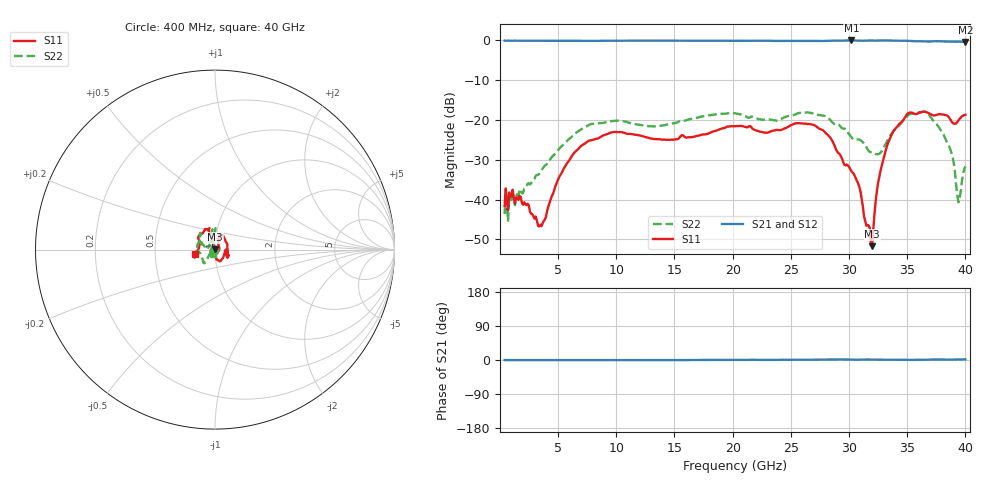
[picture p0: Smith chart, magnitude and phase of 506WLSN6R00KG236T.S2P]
!  American Technical Ceramics  Date:  8/31/2012
!  One Norden Lane
!  Huntington Station,  NY.  11746-2102
!  Tel:  (631) 622-4700  Fax:  (631) 622-4748
!  Part Number  506WLSN6R00KG236T
!  Description:  Ultra-Broadband Inductor
!  Application:  Ultra-broadband DC block decoupling, bias tee
# GHZ S DB R 50
! Freq  |S11|  S11 Ph  |S21|  S21 Ph  |S12|  S12 Ph  |S22|  S22 Ph
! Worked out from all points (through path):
!   401 points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, 400 MHz to 40 GHz, reference 50 ohm
!   highest |S21| = -0.01 dB at 30.2 GHz (marker M1); lowest = -0.4 dB at 40 GHz (marker M2)
!   lowest |S11| = -51.7 dB at 31.98 GHz (marker M3), VSWR 1.01, Z = 50.1 + j0.216 ohm
!   |S11| at or under -10 dB: start of sweep to end of sweep
!   |S22| runs from -45.3 to -17.9 dB; largest |S21 - S12| = 0.0028
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0.4  -41.57 -178.8  -0.04 -0.1  -0.04 -0.1  -43.62 177.8
1.588  -40.08 167.8  -0.07 -0.2  -0.07 -0.2  -38.92 -177.4
3.469  -46.33 -155.8  -0.09 -0.3  -0.09 -0.2  -32.93 -157.0
5.251  -33.57 -86.7  -0.10 -0.3  -0.10 -0.3  -26.72 -137.4
7.033  -26.39 -83.0  -0.12 -0.3  -0.12 -0.3  -22.22 -129.0
9.805  -23.02 -67.5  -0.08 0.0  -0.07 0.0  -20.22 -128.3
13.666  -24.83 -19.5  -0.06 -0.1  -0.06 -0.1  -21.54 -163.9
20.2  -21.55 -32.0  -0.08 0.4  -0.08 0.4  -18.30 -159.9
23.665  -22.55 25.3  -0.14 0.3  -0.14 0.4  -20.14 153.3
26.833  -21.14 73.2  -0.14 0.8  -0.14 0.9  -18.31 132.3
28.318  -24.19 71.4  -0.09 1.6  -0.09 1.6  -19.79 140.5
30.199  -32.84 -2.8  -0.01 1.1  -0.01 1.2  -24.27 163.1
30.793  -36.04 -52.5  -0.06 0.8  -0.07 0.9  -24.87 173.9
31.783  -47.14 -9.4  -0.02 1.1  -0.02 1.1  -28.02 166.2
31.981  -51.70 55.9  -0.03 1.0  -0.03 1.1  -28.09 163.2
32.575  -34.62 104.5  -0.04 1.0  -0.04 1.0  -28.53 144.8
33.466  -24.97 105.7  -0.04 0.8  -0.04 0.8  -24.24 116.8
35.05  -18.35 107.2  -0.10 0.2  -0.10 0.3  -18.88 97.0
36.535  -17.93 116.3  -0.24 0.7  -0.25 0.8  -17.91 91.4
38.614  -19.43 148.2  -0.29 1.0  -0.30 1.0  -26.71 109.1
39.406  -20.13 -175.7  -0.30 1.4  -0.32 1.4  -40.69 167.1
40  -18.68 -167.0  -0.38 1.7  -0.38 1.8  -31.68 -119.6
